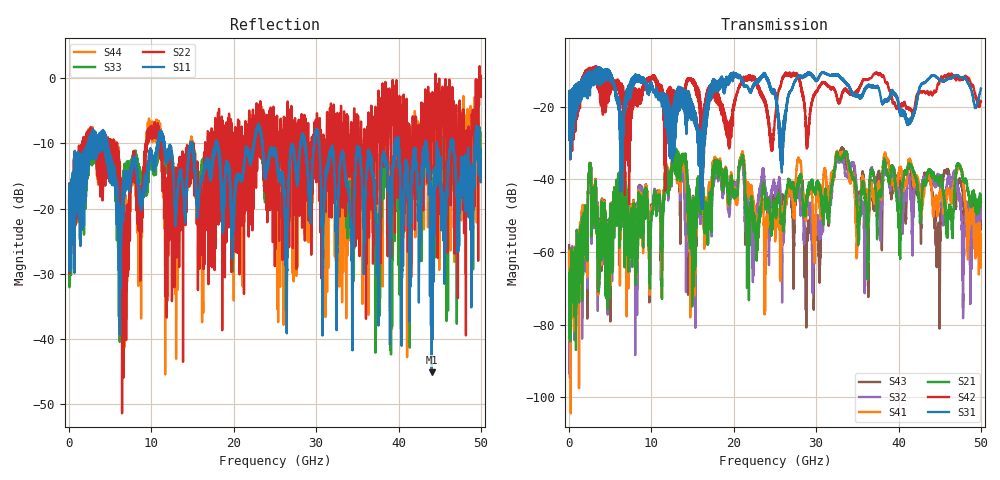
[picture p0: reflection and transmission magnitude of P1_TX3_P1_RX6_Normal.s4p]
!Keysight Technologies,N5225B,MY57041031,A.13.20.10
!Date: Friday, May 31, 2019 11:22:25
!Correction: S11(Full 4 Port(1,2,3,4))
!S12(Full 4 Port(1,2,3,4))
!S13(Full 4 Port(1,2,3,4))
!S14(Full 4 Port(1,2,3,4))
!S21(Full 4 Port(1,2,3,4))
!S22(Full 4 Port(1,2,3,4))
!S23(Full 4 Port(1,2,3,4))
!S24(Full 4 Port(1,2,3,4))
!S31(Full 4 Port(1,2,3,4))
!S32(Full 4 Port(1,2,3,4))
!S33(Full 4 Port(1,2,3,4))
!S34(Full 4 Port(1,2,3,4))
!S41(Full 4 Port(1,2,3,4))
!S42(Full 4 Port(1,2,3,4))
!S43(Full 4 Port(1,2,3,4))
!S44(Full 4 Port(1,2,3,4))
!S4P File: Measurements: <S11,S12,S13,S14>,
!<S21,S22,S23,S24>,
!<S31,S32,S33,S34>,
!<S41,S42,S43,S44>:
# Hz S  dB  R 50.0
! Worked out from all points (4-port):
!   5000 points, 10 MHz to 50 GHz, reference 50 ohm
!   strongest paths, dB at 10 MHz, 12.51 GHz, 25.01 GHz, 37.51 GHz, 50 GHz:
!     S31: -19.3, -27.1, -15.7, -14.5, -15.0
!     S42: -19.5, -15.7, -22.9, -11.0, -18.6
!     S21: -67.2, -35.3, -47.4, -48.0, -46.1
!     S41: -59.7, -34.0, -53.9, -41.4, -57.2
!     S32: -62.4, -35.8, -43.2, -45.7, -48.2
!     S43: -58.2, -34.4, -48.6, -39.3, -52.4
!   lowest |S11| = -45.1 dB at 44.03 GHz (marker M1), VSWR 1.01, Z = 49.9 + j0.541 ohm
!   |S11| at or under -10 dB: 4.66 GHz to 10.77 GHz (6.106 GHz wide, 79.2 % of centre); 23.49 GHz to 28.08 GHz (4.584 GHz wide, 17.8 % of centre); 30.37 GHz to 39.61 GHz (9.239 GHz wide, 26.4 % of centre)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
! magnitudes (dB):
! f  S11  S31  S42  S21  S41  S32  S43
! 10 MHz  -19.6  -19.3  -19.5  -67.2  -59.7  -62.4  -58.2
! 2.54 GHz  -12.5  -16.9  -11.8  -36.7  -36.5  -37.1  -36.9
! 4.65 GHz  -10.4  -11.2  -16.6  -66.9  -62.3  -64.8  -60.3
! 16.03 GHz  -15.6  -40.2  -26.5  -43.2  -46.0  -44.4  -46.6
! 19.84 GHz  -27.6  -11.3  -25.3  -41.6  -40.4  -42.2  -40.9
! 44.03 GHz  -45.1  -11.4  -16.6  -38.8  -42.9  -39.4  -42.9
! 50 GHz  -12.4  -15.0  -18.6  -46.1  -57.2  -48.2  -52.4
